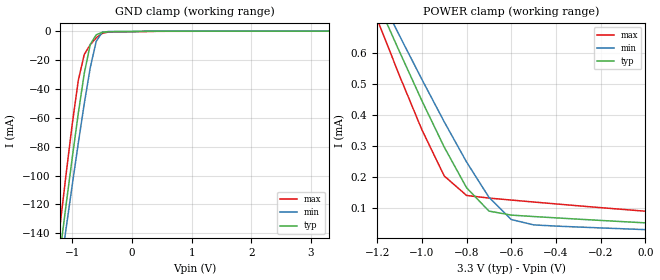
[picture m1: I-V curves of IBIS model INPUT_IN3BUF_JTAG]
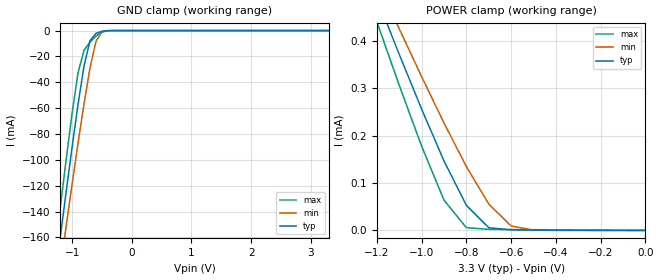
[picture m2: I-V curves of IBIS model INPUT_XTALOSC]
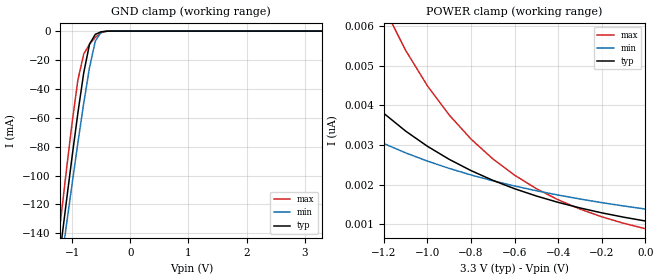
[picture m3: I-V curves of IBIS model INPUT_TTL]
| IBIS file 9885t.ibs created by s2ibis2 version 1.2
| North Carolina State University Electronics Research Laboratory  1995
[IBIS ver]   2.1
[File name]   5v9885t.ibs
[File Rev]   1.1
[Date]   Apr 13, 2012
[Source]   IDT
[Notes]   1. Temp typ=25C, min=100C, max=-40C
   2. IDT  C11.5, 3.3v process
   3. Ramp rates based on 50 ohm load
[Disclaimer]
READ THESE TERMS AND CONDITIONS CAREFULLY BEFORE USING THIS IBIS MODEL.  BY
USING THIS IBIS MODEL, YOU ARE ACCEPTING AND AGREEING TO THESE TERMS AND
CONDITIONS OF USE.
Integrated Device Technology, Inc. ("IDT") hereby grants the user of this
IBIS model ("User") a non-exclusive, nontransferable license to use this
IBIS model under the following terms: The User is granted this license only
to use the IBIS model for demonstration purposes only and is not granted
rights to sell, copy (except as needed to run the IBIS model), rent, lease
or sub-license (except for demonstration) the IBIS model in whole or in
part, or in modified form to anyone. The User may modify the IBIS model to
suit its specific applications, but  rights to derivative works and such
modifications shall belong to IDT.
THIS IBIS MODEL IS PROVIDED ON AN AS IS" BASIS AND IDT  MAKES ABSOLUTELY NO
WARRANTY WITH RESPECT TO THE INFORMATION CONTAINED HEREIN.  IDT DISCLAIMS
AND USER WAIVES ALL WARRANTIES, EXPRESS AND IMPLIED, INCLUDING WARRANTIES OF
MERCHANTABILITY AND FITNESS FOR A PARTICULAR PURPOSE.  THE ENTIRE RISK AS TO
QUALITY AND PERFORMANCE IS WITH THE USER  ACCORDINGLY, IN NO EVENT SHALL IDT
BE LIABLE FOR ANY DIRECT OR INDIRECT DAMAGES, WHETHER IN CONTRACT OR TORT,
INCLUDING ANY LOST PROFITS OR OTHER INCIDENTAL, CONSEQUENTIAL, EXEMPLARY, OR
PUNITIVE DAMAGES ARISING OUT OF THE USE OR APPLICATION OF THE  IBIS MODEL,
WHETHER OR NOT IDT HAD NOTICE OF SUCH DAMAGES.
IDT reserves the right to make changes without notice to any product herein
to improve reliability, function, or design. IDT does not convey any license
under patent rights or any other intellectual property rights, including
those of third parties. IDT is not obligated to provide  maintenance or
support for the licensed IBIS model.
This model is for  IDT5V9885T IDT Programmable Clock
[Copyright]
Copyright 2002, Integrated Device Technology, Inc. All rights  reserved.
|History
|Rev 1.0 Created on Jan 03 2012
|   Component IDT5V9885TNL
[Component]   IDT5V9885TNL
[Manufacturer]   Integrated Device Technology Inc.
[Package]
| Following package parameters are for the 28 pin QFBN package
| variable   typ   min   max
R_pkg   0.11000   60.00000m   0.15500
L_pkg   3.23000nH   1.80000nH   4.55000nH
C_pkg   0.12400pF   77.00000fF   0.16700pF
[Pin]  signal_name   model_name   R_pin   L_pin   C_pin
1   CLKIN   INPUT_XTALOSC
2   GND   GND
3   GOUT1/LOSS_CLKIN   IO_TTL
4   XTALIN/REFIN   INPUT_XTALOSC
5   OUT1   OUTPUT_TTL
6   OUT3   OUTPUT_TTL
7   XTALOUT   OUTPUT_TTL
8   OUT4   OUTPUT_TTL
9   OUT4B   OUTPUT_TTL
10   VDD   POWER
11   OUT6   OUTPUT_TTL
12   OUT5   OUTPUT_TTL
13   OUT5B   OUTPUT_TTL
14   VDD   POWER
15   GIN0/SDA/TDI   IO_TTL_SDA
16   GIN1/SCLK/TCLK   INPUT_TTL
17   GIN5/CLK_SEL   INPUT_TTL
18   I2C/JTAG   INPUT_IN3BUF_JTAG
20   VDD   POWER
21   GIN2/TMS   INPUT_TTL
22   GIN4/TRST   INPUT_TTL
23   GIN3/SUSPEND   INPUT_TTL
24   SHUTDOWN/OE   INPUT_TTL
25   OUT2   OUTPUT_TTL
26   GND   GND
27   GOUT0/TDO/LOSS_LOCK   IO_TTL
28   VDD   POWER
|   Component IDT5V9885TPF
[Component]   IDT5V9885TPF
[Manufacturer]   Integrated Device Technology Inc.
[Package]
| Following package parameters are for the 28 pin QFBN package
| variable   typ   min   max
R_pkg   0.11000   60.00000m   0.15500
L_pkg   3.23000nH   1.80000nH   4.55000nH
C_pkg   0.12400pF   77.00000fF   0.16700pF
[Pin]  signal_name   model_name   R_pin   L_pin   C_pin
1   CLKIN   INPUT_XTALOSC
2   GND   GND
3   GOUT1/LOSS_CLKIN   IO_TTL
4   XTALIN/REFIN   INPUT_XTALOSC
5   XTALOUT   OUTPUT_TTL
6   OUT1   OUTPUT_TTL
7   VDD   POWER
8   OUT3   OUTPUT_TTL
9   GND   GND
10   OUT4   OUTPUT_TTL
11   OUT4B   OUTPUT_TTL
12   VDD   POWER
13   OUT6   OUTPUT_TTL
14   VDD   POWER
15   OUT5   OUTPUT_TTL
16   OUT5B   OUTPUT_TTL
17   VDD   POWER
18   GND   GND
20   GIN1/SCLK/TCK   INPUT_TTL
21   GIN5/CLK_SEL   INPUT_TTL
22   I2C/JTAG   INPUT_IN3BUF_JTAG
23   VDD   POWER
24   GIN2/TMS   INPUT_TTL
25   GIN4/TRST   INPUT_TTL
26   GND   GND
27   GIN3/SUSPEND   INPUT_TTL
28   SHUTDOWN/OE   INPUT_TTL
29   OUT2   OUTPUT_TTL
30   GND   GND
31   GOUT0/TDO/LOSS_LOCK   IO_TTL
32   VDD   POWER
| Models and submodels in the file (6): INPUT_IN3BUF_JTAG (Input), INPUT_XTALOSC (Input), INPUT_TTL (Input), IO_TTL_SDA (I/O_open_sink), OUTPUT_TTL (3-state), IO_TTL (3-state)
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| oe   oe   dummy_model
| oe1  oe1   dummy_model
| oe2  oe2   dummy_model
| din  din   dummy_model
| d_sdad_sda   dummy_model
| en   en   dummy_model
| d_oscd_osc   dummy_model
| d   d   dummy_model
|   Model INPUT_IN3BUF_JTAG
[Model]   INPUT_IN3BUF_JTAG
Model_type   Input
Polarity   Non-Inverting
Vinl =  0.80000V
Vinh =  2.00000V
C_comp   3.15000pF   3.15000pF   3.15000pF
[Temperature Range]   25.00000   100.00000   -40.00000
[Voltage Range]   3.30000V   3.00000V   3.60000V
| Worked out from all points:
|   GND clamp passes 1 mA (typ) near -0.51 V on its own axis
|   POWER clamp passes 1 mA (typ) near -1.34 V on its own axis
[GND_clamp]
| voltage   I(typ)   I(min)   I(max)
-3.3V     -860.5mA   -813.9mA   -910.2mA
-1.3V     -183.6mA   -194.8mA   -167.8mA
-1.2V     -150.9mA   -164.8mA   -132.2mA
-1.1V     -118.6mA   -135.1mA   -97.2mA
-1V       -87.04mA   -105.9mA   -63.68mA
-900mV    -56.7mA    -77.34mA   -33.92mA
-800mV    -29.1mA    -50.04mA   -16.08mA
-700mV    -9.176mA   -25.28mA   -9.381mA
-600mV    -2.482mA   -6.996mA   -4.572mA
-500mV    -777.2uA   -845.2uA   -1.547mA
-400mV    -376uA     -257.6uA   -619.7uA
3.3V      52.22uA    38.84uA    73.56uA
[POWER_clamp]
| voltage   I(typ)   I(min)   I(max)
-3.3V     4.322mA    3.934mA    4.774mA
-1.2V     764.2uA    797.5uA    707.7uA
-1.1V     602.9uA    654.5uA    525.6uA
-1V       445.3uA    514uA      351.9uA
-900mV    296uA      377.3uA    203.1uA
-800mV    165.1uA    247.9uA    140.4uA
-700mV    90.1uA     134.5uA    132uA
-600mV    77.2uA     62.88uA    125.6uA
-500mV    72.57uA    45.75uA    119.3uA
0V        52.22uA    30.49uA    89.76uA
|   Model INPUT_XTALOSC
[Model]   INPUT_XTALOSC
Model_type   Input
Polarity   Non-Inverting
Vinl =  0.80000V
Vinh =  2.00000V
C_comp   4.00000pF   4.00000pF   4.00000pF
[Temperature Range]   25.00000   100.00000   -40.00000
[Voltage Range]   3.30000V   3.00000V   3.60000V
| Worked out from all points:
|   GND clamp passes 1 mA (typ) near -0.53 V on its own axis
|   POWER clamp passes 1 mA (typ) near -1.62 V on its own axis
[GND_clamp]
| voltage   I(typ)   I(min)   I(max)
-3.3V     -943.7mA   -911.4mA   -977.9mA
-1.3V     -196.5mA   -218.3mA   -176.1mA
-1.2V     -160.4mA   -184.7mA   -137.6mA
-1.1V     -124.9mA   -151.5mA   -99.98mA
-1V       -90.17mA   -118.9mA   -63.99mA
-900mV    -56.99mA   -87.01mA   -32.53mA
-800mV    -27.37mA   -56.54mA   -15.26mA
-700mV    -7.824mA   -28.91mA   -8.942mA
-600mV    -2.175mA   -8.303mA   -4.213mA
-500mV    -492.4uA   -874.3uA   -1.14mA
-400mV    -59.94uA   -63.48uA   -132.1uA
3.3V      67.86nA    72.43nA    13.64nA
[POWER_clamp]
| voltage   I(typ)   I(min)   I(max)
-3.3V     3.118mA    2.794mA    3.419mA
-1.2V     490.8uA    528.9uA    440.7uA
-1.1V     371.9uA    425.9uA    306.6uA
-1V       256.3uA    324.8uA    178uA
-900mV    146.8uA    227uA      63.96uA
-800mV    52.93uA    134.9uA    5.913uA
-700mV    5.782uA    55.77uA    2.388uA
-600mV    1.226uA    9.437uA    1.951uA
-500mV    889.4nA    759.8nA    1.591uA
0V        67.86nA    4.057nA    297.8nA
|   Model INPUT_TTL
[Model]   INPUT_TTL
Model_type   Input
Polarity   Non-Inverting
Vinl =  0.80000V
Vinh =  2.00000V
C_comp   3.15000pF   3.15000pF   3.15000pF
[Temperature Range]   25.00000   100.00000   -40.00000
[Voltage Range]   3.30000V   3.00000V   3.60000V
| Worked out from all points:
|   GND clamp passes 1 mA (typ) near -0.53 V on its own axis
[GND_clamp]
| voltage   I(typ)   I(min)   I(max)
-3.3V     -860.5mA   -813.9mA   -910.1mA
-1.3V     -183.6mA   -194.8mA   -167.8mA
-1.2V     -150.9mA   -164.8mA   -132.1mA
-1.1V     -118.6mA   -135.1mA   -97.13mA
-1V       -86.99mA   -105.9mA   -63.61mA
-900mV    -56.64mA   -77.31mA   -33.82mA
-800mV    -29.01mA   -50mA      -15.89mA
-700mV    -9.031mA   -25.22mA   -9.146mA
-600mV    -2.261mA   -6.881mA   -4.277mA
-500mV    -493.9uA   -650.7uA   -1.144mA
-400mV    -59.34uA   -43.85uA   -131.5uA
3.3V      1.08nA     1.636nA    591.5pA
[POWER_clamp]
| voltage   I(typ)   I(min)   I(max)
-3.3V     74.3nA     29.42nA    315.2nA
-1.9V     9.867nA    5.868nA    24.24nA
-1.6V     6.467nA    4.338nA    13.72nA
-1.5V     5.639nA    3.947nA    11.36nA
-1.4V     4.929nA    3.604nA    9.41nA
-1.2V     3.799nA    3.036nA    6.48nA
-1.1V     3.351nA    2.801nA    5.39nA
-1V       2.967nA    2.593nA    4.494nA
-900mV    2.637nA    2.408nA    3.756nA
-700mV    2.107nA    2.096nA    2.649nA
-400mV    1.55nA     1.735nA    1.615nA
0V        1.08nA     1.382nA    886.8pA
